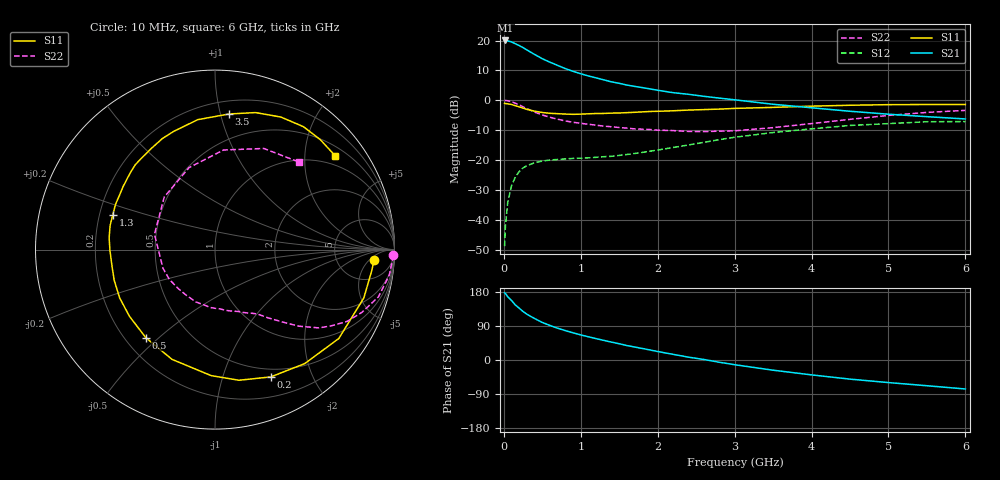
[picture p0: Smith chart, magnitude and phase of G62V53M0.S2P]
! SIEMENS Small Signal Semiconductors
! BFG193
! Si NPN RF Bipolar Junction Transistor in SOT223
! VCE = 2.5 V  IC = 3 mA
! Common Emitter S-Parameters:  August  1996
# GHz  S  MA  R  50
!  f  S11  S21  S12  S22
! GHz  MAG  ANG  MAG  ANG  MAG  ANG  MAG  ANG
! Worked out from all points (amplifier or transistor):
!   36 points, 10 MHz to 6 GHz, reference 50 ohm
!   highest |S21| = 20.0 dB at 20 MHz (marker M1)
!   |S21| within 3 dB of that: start of sweep to 287.9 MHz
!   unconditionally stable (mu >= 1): 1.272 GHz to 2.641 GHz
!   at 250 MHz: K = 0.24, MSG = 20.1 dB, |S12| = -22.7 dB
!   at 1.4 GHz: K = 1.07, MAG = 10.8 dB, |S12| = -18.8 dB
!   at 6 GHz: K = 0.94, MSG = 0.4 dB, |S12| = -7.1 dB
!   S11 on the Smith chart (normalised r, x): 10 MHz: 13, -7; 200 MHz: 0.41, -1.45; 500 MHz: 0.28, -0.45; 1.3 GHz: 0.26, +0.16; 3.5 GHz: 0.30, +1.06; 6 GHz: 0.73, +2.73
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0.01  0.8879 -3.6  9.979 177.4  0.0036 92.7  0.994 -1.8
0.02  0.8813 -7.6  10.03 175.8  0.0076 85.1  0.9902 -3.4
0.05  0.8718 -18.0  9.875 167.1  0.0193 80.2  0.9814 -8.3
0.1  0.8491 -35.7  9.474 157.0  0.0371 71.9  0.9479 -16.1
0.15  0.8083 -51.8  8.843 145.1  0.0518 62.5  0.8904 -23.1
0.2  0.7742 -66.4  8.23 136.6  0.0641 56.1  0.838 -28.5
0.25  0.7401 -79.6  7.603 127.9  0.0737 50.1  0.774 -33.3
0.3  0.7026 -91.7  6.949 120.8  0.0803 45.4  0.725 -37.0
0.4  0.6568 -111.4  5.848 109.4  0.09 38.3  0.6328 -42.4
0.5  0.6239 -128.2  4.959 99.1  0.0957 32.9  0.5663 -46.1
0.6  0.6044 -142.0  4.333 91.1  0.0999 30.2  0.5188 -49.2
0.7  0.5956 -153.2  3.829 83.9  0.102 27.9  0.4811 -52.2
0.9  0.5811 -171.2  3.055 71.7  0.1061 25.9  0.4278 -56.9
1.1  0.5933 173.7  2.551 61.2  0.1086 26.1  0.3955 -63.1
1.3  0.6015 161.2  2.193 51.7  0.1134 27.2  0.3685 -69.2
1.6  0.6205 145.7  1.795 38.1  0.1235 29.2  0.3416 -81.1
2.2  0.6662 122.1  1.34 14.9  0.1618 30.4  0.3105 -109.9
2.8  0.7107 103.1  1.087 -5.9  0.2187 24.7  0.3036 -147.0
3.5  0.7596 84.1  0.856 -26.9  0.2881 10.5  0.3479 165.7
4.5  0.8246 63.6  0.654 -50.5  0.3784 -11.5  0.4791 107.6
5.5  0.8482 46.3  0.531 -67.9  0.4367 -38.5  0.6258 64.2
6  0.8496 38.0  0.486 -76.5  0.4398 -53.2  0.6768 46.0
